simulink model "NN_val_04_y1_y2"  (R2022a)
settings: Solver=VariableStepAuto  StartTime=0.0  StopTime=300  RelTol=1e-3
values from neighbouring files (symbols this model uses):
  C = 6.3000e-04    (= 0.00063)    [maglev_init.m]
  g = 9.80    (= 9.8)    [maglev_init.m]
  K = 1.0e+03 * [-2.4567   -0.1235    0.0237]    [maglev_init.m]
  L1 = 0.6000    (= 0.6)    [maglev_init.m]
  m = 0.0300    (= 0.03)    [maglev_init.m]
  mpert = 0    [maglev_init.m]
  R = 45    [maglev_init.m]
  Ts = 0.005    [maglev_init.m]    (also in train_net.m)
  x1_0 = 0.1    [maglev_init.m]
  x1_d = 0.05    [maglev_init.m]
  x2_0 = 0    [maglev_init.m]
  x2_d = 0    [maglev_init.m]
  x3_0 = 0.2    [maglev_init.m]
undefined symbols (not defined in the file or in its folder): magnitude
libraries: neural x24

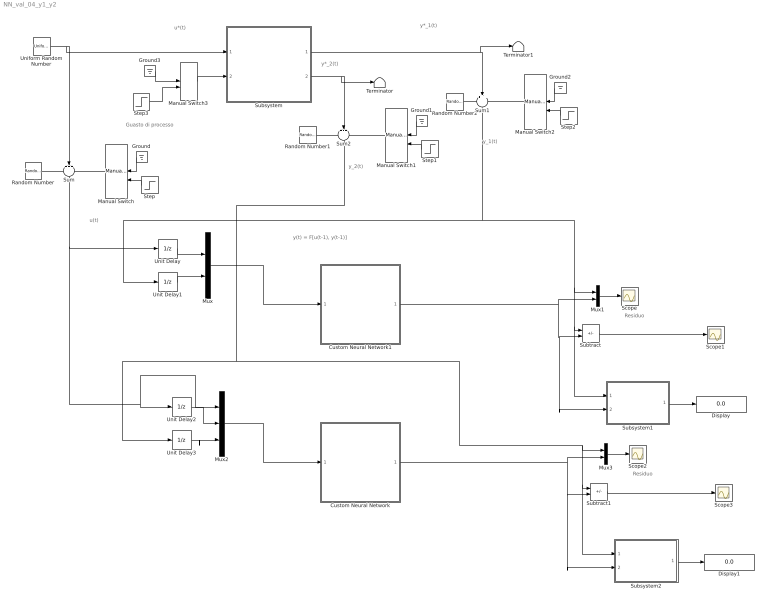
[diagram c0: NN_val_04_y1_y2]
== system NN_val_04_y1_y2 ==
  note: Residuo
  note: y(t) = F[u(t-1), y(t-1)]
  note: y_2(t)
  note: y*_1(t)
  note: u(t)
  note: y*_2(t)
  note: y_1(t)
  note: u*(t)
  note: Guasto di processo
  note: Residuo
  Custom Neural Network : Subsystem
      mask help: Custom Neural Network
  Custom Neural Network1 : Subsystem
      mask help: Custom Neural Network
  Display : Display
  Display1 : Display
  Ground{,1..3} (4 alike) : Ground
  Manual Switch : ManualSwitch
  Manual Switch1 : ManualSwitch  CurrentSetting=0
  Manual Switch2 : ManualSwitch
  Manual Switch3 : ManualSwitch
  Mux : Mux  Inputs=2
  Mux1 : Mux  Inputs=2
  Mux2 : Mux  Inputs=3
  Mux3 : Mux  Inputs=2
  Random Number : RandomNumber  Variance=1e-9  Seed=1  SampleTime=Ts
  Random Number1 : RandomNumber  Variance=1e-6  Seed=3  SampleTime=Ts
  Random Number2 : RandomNumber  Variance=1e-9  Seed=2  SampleTime=Ts
  Scope{,1..3} (4 alike) : Scope
  Step : Step  Time=150  SampleTime=0
  Step1 : Step  Time=150  SampleTime=0
  Step2 : Step  Time=150  SampleTime=0
  Step3 : Step  Time=15  After=2*R  SampleTime=0
  Subsystem : Subsystem
  Subsystem1 : Subsystem
  Subsystem2 : Subsystem
  Subtract : Sum  Inputs=+-
  Subtract1 : Sum  Inputs=+-
  Sum : Sum  Inputs=+++
  Sum1 : Sum  Inputs=+++
  Sum2 : Sum  Inputs=+++
  Terminator : Terminator
  Terminator1 : Terminator
  Uniform Random Number : UniformRandomNumber  Minimum=x1_d*0.9  Maximum=x1_d*1.1  Seed=1  SampleTime=0.5
  Unit Delay{,1..3} (4 alike) : UnitDelay  SampleTime=Ts  HasFrameUpgradeWarning=on
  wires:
  Subsystem/1(Out1) -> Terminator1/1, Sum1/2
  Subsystem/2(Out2) -> Terminator/1, Sum2/2
  Random Number/1 -> Sum/1
  Manual Switch/1 -> Sum/3
  Manual Switch2/1 -> Sum1/3
  Manual Switch1/1 -> Sum2/3
  Random Number1/1 -> Sum2/1
  Ground/1 -> Manual Switch/1
  Step/1 -> Manual Switch/2
  Ground1/1 -> Manual Switch1/1
  Step1/1 -> Manual Switch1/2
  Random Number2/1 -> Sum1/1
  Ground2/1 -> Manual Switch2/1
  Step2/1 -> Manual Switch2/2
  Manual Switch3/1 -> Subsystem/2(fs)
  Ground3/1 -> Manual Switch3/1
  Uniform Random Number/1 -> Subsystem/1(u), Sum/2
  Step3/1 -> Manual Switch3/2
  Sum/1 -> Mux2/1, Unit Delay2/1, Unit Delay/1
  Unit Delay/1 -> Mux/1
  Unit Delay1/1 -> Mux/2
  Mux/1 -> Custom Neural Network1/1(Input)
  Custom Neural Network1/1(Output) -> Mux1/2, Subsystem1/2(y_prev), Subtract/2
  Subtract/1 -> Scope1/1
  Mux1/1 -> Scope/1
  Sum1/1 -> Subsystem1/1(y_mis), Subtract/1, Mux1/1, Unit Delay1/1
  Subsystem1/1(VAF%) -> Display/1
  Mux2/1 -> Custom Neural Network/1(Input)
  Unit Delay2/1 -> Mux2/2
  Unit Delay3/1 -> Mux2/3
  Subtract1/1 -> Scope3/1
  Custom Neural Network/1(Output) -> Mux3/2, Subsystem2/2(y_prev), Subtract1/2
  Mux3/1 -> Scope2/1
  Subsystem2/1(VAF%) -> Display1/1
  Sum2/1 -> Subsystem2/1(y_mis), Subtract1/1, Mux3/1, Unit Delay3/1

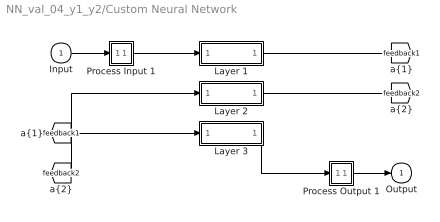
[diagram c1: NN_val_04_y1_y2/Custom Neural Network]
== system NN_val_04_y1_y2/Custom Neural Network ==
  Input : Inport  PortDimensions=3  SampleTime=0.005
  Layer 1 : Subsystem
  Layer 2 : Subsystem
  Layer 3 : Subsystem
  Process Input 1 : Subsystem
  Process Output 1 : Subsystem
  Output : Outport  InitialOutput=0
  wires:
  Input/1 -> Process Input 1/1(x)
  Process Output 1/1(y) -> Output/1
  Process Input 1/1(p) -> Layer 1/1("p{1}")
  Layer 1/1("a{1}") -> [feedback1]
  [feedback1] -> Layer 2/1("a{1} ")
  Layer 2/1("a{2}") -> [feedback2]
  [feedback2] -> Layer 3/1("a{2} ")
  Layer 3/1("a{3}") -> Process Output 1/1(a)

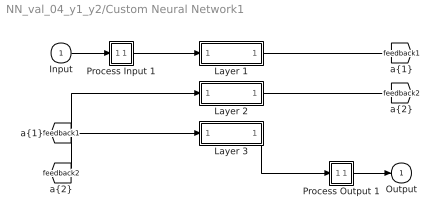
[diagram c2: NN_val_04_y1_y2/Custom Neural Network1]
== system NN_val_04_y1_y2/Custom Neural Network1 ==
  Input : Inport  PortDimensions=2  SampleTime=0.005
  Layer 1 : Subsystem
  Layer 2 : Subsystem
  Layer 3 : Subsystem
  Process Input 1 : Subsystem
  Process Output 1 : Subsystem
  Output : Outport  InitialOutput=0
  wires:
  Layer 3/1("a{3}") -> Process Output 1/1(a)
  [feedback2] -> Layer 3/1("a{2} ")
  Layer 2/1("a{2}") -> [feedback2]
  [feedback1] -> Layer 2/1("a{1} ")
  Layer 1/1("a{1}") -> [feedback1]
  Process Input 1/1(p) -> Layer 1/1("p{1}")
  Process Output 1/1(y) -> Output/1
  Input/1 -> Process Input 1/1(x)

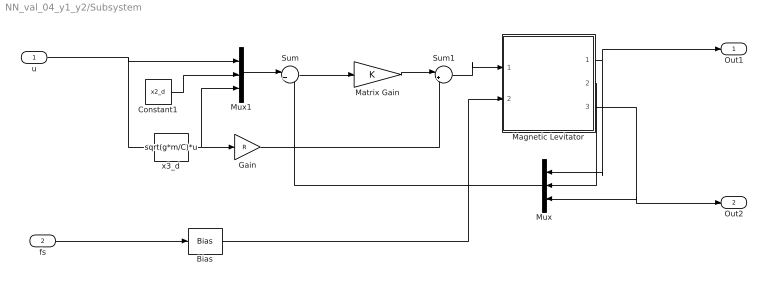
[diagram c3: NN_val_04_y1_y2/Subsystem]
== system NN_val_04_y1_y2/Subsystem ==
  u : Inport
  fs : Inport  Port=2
  Bias : Bias  Bias=R
  Constant1 : Constant  Value=x2_d
  Gain : Gain  Gain=R
  Magnetic Levitator : Subsystem  mask{m=m+mpert, R=R, L1=L1, C=C, g=g}
      mask prompts: m "ball's mass (m)"; R "Electromagnet's resistance (R)"; L1 "Electromagnet's inductance (L1)"; C "Magnetic force constant (C)"; g "Gravitational acceleration (g)"
  Matrix Gain : Gain  Gain=K  Multiplication=Matrix(K*u)  SaturateOnIntegerOverflow=on
  Mux : Mux  Inputs=3
  Mux1 : Mux  Inputs=3
  Sum : Sum  Inputs=|+-  InputSameDT=on  SaturateOnIntegerOverflow=on
  Sum1 : Sum  Inputs=|++  InputSameDT=on  SaturateOnIntegerOverflow=on
  x3_d : Fcn  Expr=sqrt(g*m/C)*u
  Out1 : Outport
  Out2 : Outport  Port=2
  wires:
  u/1 -> x3_d/1, Mux1/1
  Magnetic Levitator/2(x2) -> Mux/2
  x3_d/1 -> Mux1/3, Gain/1
  Mux1/1 -> Sum/1
  Gain/1 -> Sum1/2
  Mux/1 -> Sum/2
  Constant1/1 -> Mux1/2
  Sum/1 -> Matrix Gain/1
  Sum1/1 -> Magnetic Levitator/1(u)
  Magnetic Levitator/1(x1) -> Out1/1, Mux/1
  Magnetic Levitator/3(x3) -> Out2/1, Mux/3
  Matrix Gain/1 -> Sum1/1
  Bias/1 -> Magnetic Levitator/2(fs)
  fs/1 -> Bias/1

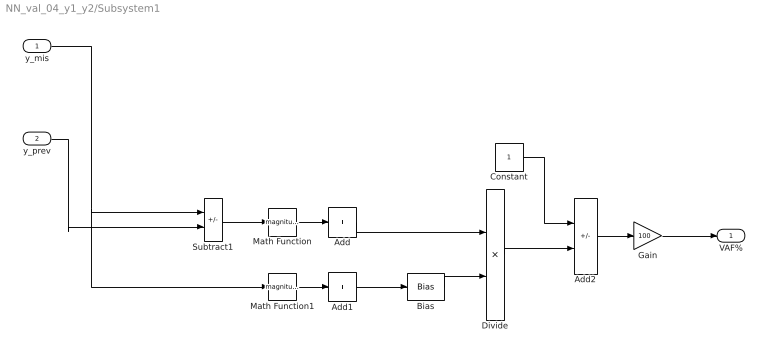
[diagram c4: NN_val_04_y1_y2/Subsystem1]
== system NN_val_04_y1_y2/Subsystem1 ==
  y_mis : Inport
  y_prev : Inport  Port=2
  Add : Sum  Inputs=+
  Add1 : Sum  Inputs=+
  Add2 : Sum  Inputs=+-
  Bias : Bias  Bias=1e-7
  Constant : Constant
  Divide : Product  Inputs=*/
  Gain : Gain  Gain=100
  Math Function : Math  Operator=magnitude^2
  Math Function1 : Math  Operator=magnitude^2
  Subtract1 : Sum  Inputs=+-
  VAF% : Outport
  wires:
  Add2/1 -> Gain/1
  Math Function/1 -> Add/1
  Bias/1 -> Divide/2
  y_mis/1 -> Math Function1/1, Subtract1/1
  Add1/1 -> Bias/1
  Math Function1/1 -> Add1/1
  Subtract1/1 -> Math Function/1
  Constant/1 -> Add2/1
  Divide/1 -> Add2/2
  Add/1 -> Divide/1
  y_prev/1 -> Subtract1/2
  Gain/1 -> VAF%/1

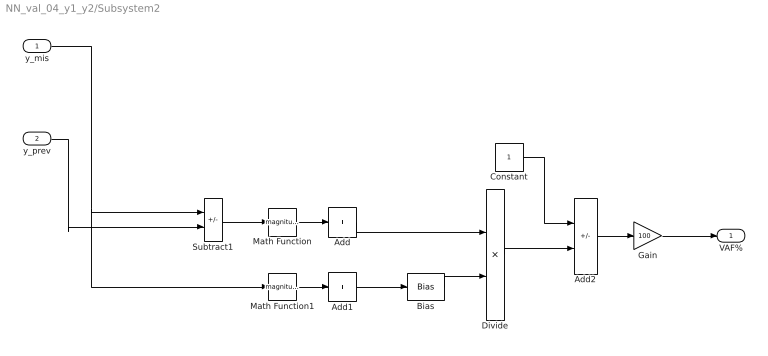
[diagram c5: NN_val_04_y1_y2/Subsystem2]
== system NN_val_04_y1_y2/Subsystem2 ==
  y_mis : Inport
  y_prev : Inport  Port=2
  Add : Sum  Inputs=+
  Add1 : Sum  Inputs=+
  Add2 : Sum  Inputs=+-
  Bias : Bias  Bias=1e-7
  Constant : Constant
  Divide : Product  Inputs=*/
  Gain : Gain  Gain=100
  Math Function : Math  Operator=magnitude^2
  Math Function1 : Math  Operator=magnitude^2
  Subtract1 : Sum  Inputs=+-
  VAF% : Outport
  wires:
  Add2/1 -> Gain/1
  Math Function/1 -> Add/1
  Bias/1 -> Divide/2
  y_mis/1 -> Math Function1/1, Subtract1/1
  Add1/1 -> Bias/1
  Math Function1/1 -> Add1/1
  Subtract1/1 -> Math Function/1
  Constant/1 -> Add2/1
  Divide/1 -> Add2/2
  Add/1 -> Divide/1
  y_prev/1 -> Subtract1/2
  Gain/1 -> VAF%/1

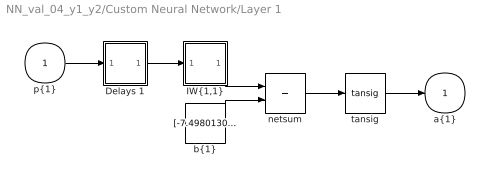
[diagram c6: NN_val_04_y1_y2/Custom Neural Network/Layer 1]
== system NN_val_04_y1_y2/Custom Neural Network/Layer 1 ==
  "p{1}" : Inport  PortDimensions=3  SampleTime=0.005
  Delays 1 : Subsystem
  "IW{1,1}" : Subsystem
  "b{1}" : Constant  Value=[-7.49801301032872391516548304934985935688018798828125;-8.469632793028239348132046870887279510498046875;-6.44515742607553843157575101940892636775970458984375]
  netsum : Sum  Inputs=2  InputSameDT=on  SaturateOnIntegerOverflow=on
  tansig : neural/Transfer Functions/tansig
  "a{1}" : Outport  InitialOutput=[0;0;0]
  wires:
  "p{1}"/1 -> Delays 1/1("p{1}")
  Delays 1/1("pd{1,1}") -> "IW{1,1}"/1("pd{1,1}")
  "IW{1,1}"/1("iz{1,1}") -> netsum/1
  "b{1}"/1 -> netsum/2
  netsum/1 -> tansig/1
  tansig/1 -> "a{1}"/1

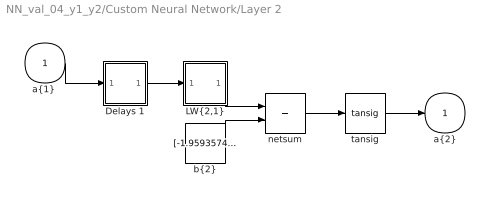
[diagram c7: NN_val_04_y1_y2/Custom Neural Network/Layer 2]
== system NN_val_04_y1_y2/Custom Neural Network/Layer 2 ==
  "a{1} " : Inport  PortDimensions=3  SampleTime=0.005
  Delays 1 : Subsystem
  "LW{2,1}" : Subsystem
  "b{2}" : Constant  Value=[-1.9593574661046309071110727018094621598720550537109375;-1.733772264384629835376472328789532184600830078125;-1.2022508025021882982485976754105649888515472412109375;0.15838977813118992887808644809410907328128814697265625;-0.346755044752183161360648000481887720525264739990234375;-1.1898913744646983925434824413969181478023529052734375;3.4402368274347878696062252856791019439697265625]
  netsum : Sum  Inputs=2  InputSameDT=on  SaturateOnIntegerOverflow=on
  tansig : neural/Transfer Functions/tansig
  "a{2}" : Outport  InitialOutput=[0;0;0;0;0;0;0]
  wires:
  "a{1} "/1 -> Delays 1/1("p{2}")
  Delays 1/1("pd{2,1}") -> "LW{2,1}"/1("ad{2,1}")
  "LW{2,1}"/1("lz{2,1}") -> netsum/1
  "b{2}"/1 -> netsum/2
  netsum/1 -> tansig/1
  tansig/1 -> "a{2}"/1

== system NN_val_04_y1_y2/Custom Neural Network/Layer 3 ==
  "a{2} " : Inport  PortDimensions=7  SampleTime=0.005
  Delays 1 : Subsystem
  "LW{3,2}" : Subsystem
  "b{3}" : Constant  Value=0.6308795893444221203338884151889942586421966552734375
  netsum : Sum  Inputs=2  InputSameDT=on  SaturateOnIntegerOverflow=on
  purelin : neural/Transfer Functions/purelin
  "a{3}" : Outport  InitialOutput=0
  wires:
  "a{2} "/1 -> Delays 1/1("p{3}")
  Delays 1/1("pd{3,2}") -> "LW{3,2}"/1("ad{3,2}")
  "LW{3,2}"/1("lz{3,2}") -> netsum/1
  "b{3}"/1 -> netsum/2
  netsum/1 -> purelin/1
  purelin/1 -> "a{3}"/1

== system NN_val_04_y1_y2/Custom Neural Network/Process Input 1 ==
  x : Inport  PortDimensions=3  SampleTime=0.005
  p : Outport  PortDimensions=3  SampleTime=0.005
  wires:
  x/1 -> p/1

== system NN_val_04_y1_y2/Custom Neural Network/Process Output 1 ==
  a : Inport  PortDimensions=1  SampleTime=0.005
  y : Outport  PortDimensions=1  SampleTime=0.005
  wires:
  a/1 -> y/1

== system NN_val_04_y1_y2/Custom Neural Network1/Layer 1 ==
  "p{1}" : Inport  PortDimensions=2  SampleTime=0.005
  Delays 1 : Subsystem
  "IW{1,1}" : Subsystem
  "b{1}" : Constant  Value=[-2.165010232984565075042837634100578725337982177734375;-0.99018084463472033629471980020753107964992523193359375]
  netsum : Sum  Inputs=2  InputSameDT=on  SaturateOnIntegerOverflow=on
  tansig : neural/Transfer Functions/tansig
  "a{1}" : Outport  InitialOutput=[0;0]
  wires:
  tansig/1 -> "a{1}"/1
  netsum/1 -> tansig/1
  "b{1}"/1 -> netsum/2
  "IW{1,1}"/1("iz{1,1}") -> netsum/1
  Delays 1/1("pd{1,1}") -> "IW{1,1}"/1("pd{1,1}")
  "p{1}"/1 -> Delays 1/1("p{1}")

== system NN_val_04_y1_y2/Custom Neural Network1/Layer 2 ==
  "a{1} " : Inport  PortDimensions=2  SampleTime=0.005
  Delays 1 : Subsystem
  "LW{2,1}" : Subsystem
  "b{2}" : Constant  Value=[-2.76409742947160541604034733609296381473541259765625;0.91391405324340713178798978333361446857452392578125;-0.79693396570784413857069239384145475924015045166015625;2.83340357653886432132139816530980169773101806640625]
  netsum : Sum  Inputs=2  InputSameDT=on  SaturateOnIntegerOverflow=on
  tansig : neural/Transfer Functions/tansig
  "a{2}" : Outport  InitialOutput=[0;0;0;0]
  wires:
  tansig/1 -> "a{2}"/1
  netsum/1 -> tansig/1
  "b{2}"/1 -> netsum/2
  "LW{2,1}"/1("lz{2,1}") -> netsum/1
  Delays 1/1("pd{2,1}") -> "LW{2,1}"/1("ad{2,1}")
  "a{1} "/1 -> Delays 1/1("p{2}")

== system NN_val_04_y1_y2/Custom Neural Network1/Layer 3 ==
  "a{2} " : Inport  PortDimensions=4  SampleTime=0.005
  Delays 1 : Subsystem
  "LW{3,2}" : Subsystem
  "b{3}" : Constant  Value=0.2010605623167778244209102922468446195125579833984375
  netsum : Sum  Inputs=2  InputSameDT=on  SaturateOnIntegerOverflow=on
  purelin : neural/Transfer Functions/purelin
  "a{3}" : Outport  InitialOutput=0
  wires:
  purelin/1 -> "a{3}"/1
  netsum/1 -> purelin/1
  "b{3}"/1 -> netsum/2
  "LW{3,2}"/1("lz{3,2}") -> netsum/1
  Delays 1/1("pd{3,2}") -> "LW{3,2}"/1("ad{3,2}")
  "a{2} "/1 -> Delays 1/1("p{3}")

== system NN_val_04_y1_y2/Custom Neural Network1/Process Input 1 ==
  x : Inport  PortDimensions=2  SampleTime=0.005
  p : Outport  PortDimensions=2  SampleTime=0.005
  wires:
  x/1 -> p/1

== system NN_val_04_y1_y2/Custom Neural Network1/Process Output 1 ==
  a : Inport  PortDimensions=1  SampleTime=0.005
  y : Outport  PortDimensions=1  SampleTime=0.005
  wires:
  a/1 -> y/1

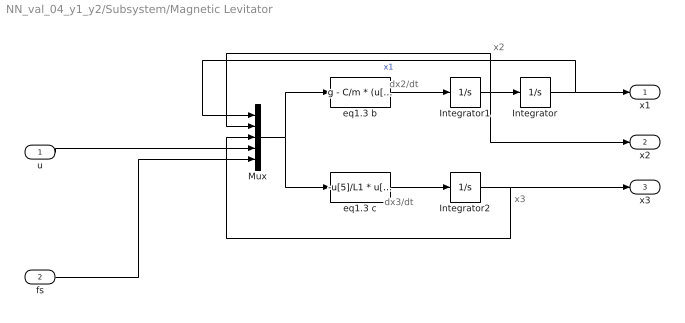
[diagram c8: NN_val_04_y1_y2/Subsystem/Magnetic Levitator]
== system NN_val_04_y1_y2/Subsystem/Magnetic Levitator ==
  note: x2
  note: x3
  note: dx2/dt
  note: dx3/dt
  u : Inport
  fs : Inport  Port=2
  Integrator : Integrator  InitialCondition=x1_0
  Integrator1 : Integrator  InitialCondition=x2_0
  Integrator2 : Integrator  InitialCondition=x3_0
  Mux : Mux  Inputs=5
  eq1.3 b : Fcn  Expr=g - C/m * (u[3] / u[1])^2
  eq1.3 c : Fcn  Expr=-u[5]/L1 * u[3] + (2*C)/L1 * ( u[2] * u[3] / u[1]^2 ) + 1/L1 * u[4]
  x1 : Outport
  x2 : Outport  Port=2
  x3 : Outport  Port=3
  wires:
  eq1.3 b/1 -> Integrator1/1
  Integrator1/1 -> Integrator/1, Mux/2, x2/1
  eq1.3 c/1 -> Integrator2/1
  Mux/1 -> eq1.3 b/1, eq1.3 c/1
  Integrator/1 -> Mux/1, x1/1  "x1"
  Integrator2/1 -> Mux/3, x3/1
  u/1 -> Mux/4
  fs/1 -> Mux/5

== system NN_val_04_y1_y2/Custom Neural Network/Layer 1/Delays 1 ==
  "p{1}" : Inport  PortDimensions=3  SampleTime=0.005
  mux : Mux  Inputs=1
  "pd{1,1}" : Outport
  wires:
  "p{1}"/1 -> mux/1
  mux/1 -> "pd{1,1}"/1

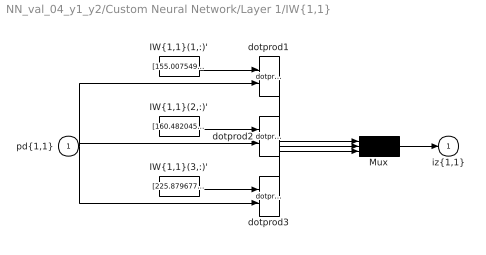
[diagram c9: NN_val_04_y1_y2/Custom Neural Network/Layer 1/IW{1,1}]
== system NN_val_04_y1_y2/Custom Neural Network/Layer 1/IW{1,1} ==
  "pd{1,1}" : Inport  PortDimensions=3  SampleTime=0.005
  "IW{1,1}(1,:)'" : Constant  Value=[155.0075492278721185357426293194293975830078125;-67.6206153138385843703872524201869964599609375;-1.56484201084633678391355715575627982616424560546875]
  "IW{1,1}(2,:)'" : Constant  Value=[160.482045237883454547045403160154819488525390625;-62.3839210025603989606679533608257770538330078125;3.692954814299637344987559117726050317287445068359375]
  "IW{1,1}(3,:)'" : Constant  Value=[225.879677595525521383024170063436031341552734375;-54.79104188249477402905540657229721546173095703125;-1.4456599193376373779784671569359488785266876220703125]
  Mux : Mux  Inputs=3
  dotprod1 : neural/Weight Functions/dotprod
  dotprod2 : neural/Weight Functions/dotprod
  dotprod3 : neural/Weight Functions/dotprod
  "iz{1,1}" : Outport
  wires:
  "IW{1,1}(1,:)'"/1 -> dotprod1/1
  "pd{1,1}"/1 -> dotprod1/2, dotprod2/2, dotprod3/2
  dotprod1/1 -> Mux/1
  "IW{1,1}(2,:)'"/1 -> dotprod2/1
  dotprod2/1 -> Mux/2
  "IW{1,1}(3,:)'"/1 -> dotprod3/1
  dotprod3/1 -> Mux/3
  Mux/1 -> "iz{1,1}"/1

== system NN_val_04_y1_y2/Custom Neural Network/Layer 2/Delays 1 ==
  "p{2}" : Inport  PortDimensions=3  SampleTime=0.005
  mux : Mux  Inputs=1
  "pd{2,1}" : Outport
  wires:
  "p{2}"/1 -> mux/1
  mux/1 -> "pd{2,1}"/1

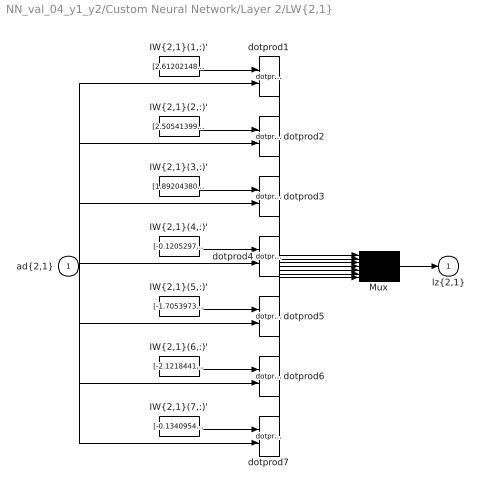
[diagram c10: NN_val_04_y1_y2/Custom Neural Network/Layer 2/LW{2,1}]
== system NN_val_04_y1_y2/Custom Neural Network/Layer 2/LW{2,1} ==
  "ad{2,1}" : Inport  PortDimensions=3  SampleTime=0.005
  "IW{2,1}(1,:)'" : Constant  Value=[2.61202148304921966115443865419365465641021728515625;0.14862508312520861242234104793169535696506500244140625;2.66275173354789185253821415244601666927337646484375]
  "IW{2,1}(2,:)'" : Constant  Value=[2.505413996791865383073627526755444705486297607421875;-0.87551618416646681541948282756493426859378814697265625;-0.4467990015803449121989388004294596612453460693359375]
  "IW{2,1}(3,:)'" : Constant  Value=[1.8920438003690247530386159269255585968494415283203125;-2.18523469881069587472666171379387378692626953125;0.99273270475465125173286651261150836944580078125]
  "IW{2,1}(4,:)'" : Constant  Value=[-0.12052978882303892749217055779809015803039073944091796875;-1.505868112384237900158723277854733169078826904296875;-0.009347378292273882116614203141580219380557537078857421875]
  "IW{2,1}(5,:)'" : Constant  Value=[-1.70539739975583959363802932784892618656158447265625;-2.30803401714740186179142256150953471660614013671875;0.43818271298305833116870644516893662512302398681640625]
  "IW{2,1}(6,:)'" : Constant  Value=[-2.12184410470687101479825287242420017719268798828125;-0.95495157641803307679850831846124492585659027099609375;0.1571940959909395030269507742559653706848621368408203125]
  "IW{2,1}(7,:)'" : Constant  Value=[-0.1340954916262217244682375394404516555368900299072265625;-0.33392737163233976449561168919899500906467437744140625;2.924572272947035589396591603872366249561309814453125]
  Mux : Mux  Inputs=7
  dotprod{1..7} (7 alike) : neural/Weight Functions/dotprod
  "lz{2,1}" : Outport
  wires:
  "IW{2,1}(1,:)'"/1 -> dotprod1/1
  "ad{2,1}"/1 -> dotprod1/2, dotprod2/2, dotprod3/2, dotprod4/2, dotprod5/2, dotprod6/2, dotprod7/2
  dotprod1/1 -> Mux/1
  "IW{2,1}(2,:)'"/1 -> dotprod2/1
  dotprod2/1 -> Mux/2
  "IW{2,1}(3,:)'"/1 -> dotprod3/1
  dotprod3/1 -> Mux/3
  "IW{2,1}(4,:)'"/1 -> dotprod4/1
  dotprod4/1 -> Mux/4
  "IW{2,1}(5,:)'"/1 -> dotprod5/1
  dotprod5/1 -> Mux/5
  "IW{2,1}(6,:)'"/1 -> dotprod6/1
  dotprod6/1 -> Mux/6
  "IW{2,1}(7,:)'"/1 -> dotprod7/1
  dotprod7/1 -> Mux/7
  Mux/1 -> "lz{2,1}"/1

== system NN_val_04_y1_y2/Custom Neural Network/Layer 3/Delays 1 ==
  "p{3}" : Inport  PortDimensions=7  SampleTime=0.005
  mux : Mux  Inputs=1
  "pd{3,2}" : Outport
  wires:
  "p{3}"/1 -> mux/1
  mux/1 -> "pd{3,2}"/1

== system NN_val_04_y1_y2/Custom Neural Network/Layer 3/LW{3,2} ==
  "ad{3,2}" : Inport  PortDimensions=7  SampleTime=0.005
  "IW{3,2}(1,:)'" : Constant  Value=[-2.790612652168341423219999342109076678752899169921875;-0.8765399083285443371238443432957865297794342041015625;0.59844685053375357153271352217416279017925262451171875;0.355938703295180236541028762076166458427906036376953125;0.46820214887316835561392736053676344454288482666015625;-2.2275650588955588915496264235116541385650634765625;-1.5266001776393240962903519175597466528415679931640625]
  Mux : Mux  Inputs=1
  dotprod1 : neural/Weight Functions/dotprod
  "lz{3,2}" : Outport
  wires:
  "IW{3,2}(1,:)'"/1 -> dotprod1/1
  "ad{3,2}"/1 -> dotprod1/2
  dotprod1/1 -> Mux/1
  Mux/1 -> "lz{3,2}"/1

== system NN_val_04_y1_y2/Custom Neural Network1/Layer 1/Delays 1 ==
  "p{1}" : Inport  PortDimensions=2  SampleTime=0.005
  mux : Mux  Inputs=1
  "pd{1,1}" : Outport
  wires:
  mux/1 -> "pd{1,1}"/1
  "p{1}"/1 -> mux/1

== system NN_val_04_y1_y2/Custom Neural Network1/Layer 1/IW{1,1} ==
  "pd{1,1}" : Inport  PortDimensions=2  SampleTime=0.005
  "IW{1,1}(1,:)'" : Constant  Value=[46.38752532641807846403025905601680278778076171875;-30.02020716206245509738437249325215816497802734375]
  "IW{1,1}(2,:)'" : Constant  Value=[50.408506029134514392353594303131103515625;28.00458439829532153453328646719455718994140625]
  Mux : Mux  Inputs=2
  dotprod1 : neural/Weight Functions/dotprod
  dotprod2 : neural/Weight Functions/dotprod
  "iz{1,1}" : Outport
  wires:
  Mux/1 -> "iz{1,1}"/1
  dotprod2/1 -> Mux/2
  "IW{1,1}(2,:)'"/1 -> dotprod2/1
  dotprod1/1 -> Mux/1
  "pd{1,1}"/1 -> dotprod2/2, dotprod1/2
  "IW{1,1}(1,:)'"/1 -> dotprod1/1

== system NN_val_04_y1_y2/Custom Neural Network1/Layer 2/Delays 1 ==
  "p{2}" : Inport  PortDimensions=2  SampleTime=0.005
  mux : Mux  Inputs=1
  "pd{2,1}" : Outport
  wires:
  mux/1 -> "pd{2,1}"/1
  "p{2}"/1 -> mux/1

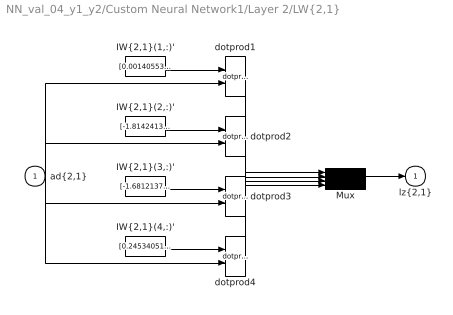
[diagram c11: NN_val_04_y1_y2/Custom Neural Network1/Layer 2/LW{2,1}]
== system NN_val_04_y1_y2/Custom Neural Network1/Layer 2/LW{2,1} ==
  "ad{2,1}" : Inport  PortDimensions=2  SampleTime=0.005
  "IW{2,1}(1,:)'" : Constant  Value=[0.001405533007920074795027431946436990983784198760986328125;2.76441434699151766807290186989121139049530029296875]
  "IW{2,1}(2,:)'" : Constant  Value=[-1.8142413042354241792253333187545649707317352294921875;2.12830136073460085555097975884564220905303955078125]
  "IW{2,1}(3,:)'" : Constant  Value=[-1.6812137832937150694334604850155301392078399658203125;-2.2096304124726291462366134510375559329986572265625]
  "IW{2,1}(4,:)'" : Constant  Value=[0.245340519136751533668672209387295879423618316650390625;2.76382363851122736519982936442829668521881103515625]
  Mux : Mux
  dotprod{1..4} (4 alike) : neural/Weight Functions/dotprod
  "lz{2,1}" : Outport
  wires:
  Mux/1 -> "lz{2,1}"/1
  dotprod4/1 -> Mux/4
  "IW{2,1}(4,:)'"/1 -> dotprod4/1
  dotprod3/1 -> Mux/3
  "IW{2,1}(3,:)'"/1 -> dotprod3/1
  dotprod2/1 -> Mux/2
  "IW{2,1}(2,:)'"/1 -> dotprod2/1
  dotprod1/1 -> Mux/1
  "ad{2,1}"/1 -> dotprod4/2, dotprod3/2, dotprod2/2, dotprod1/2
  "IW{2,1}(1,:)'"/1 -> dotprod1/1

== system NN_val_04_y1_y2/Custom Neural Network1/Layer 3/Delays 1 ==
  "p{3}" : Inport  PortDimensions=4  SampleTime=0.005
  mux : Mux  Inputs=1
  "pd{3,2}" : Outport
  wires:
  mux/1 -> "pd{3,2}"/1
  "p{3}"/1 -> mux/1

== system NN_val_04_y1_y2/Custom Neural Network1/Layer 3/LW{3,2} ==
  "ad{3,2}" : Inport  PortDimensions=4  SampleTime=0.005
  "IW{3,2}(1,:)'" : Constant  Value=[0.483295609205659226770279701668187044560909271240234375;0.356104986175123150449195463806972838938236236572265625;0.2319393811096205626487432027715840376913547515869140625;-0.2873034152097859728058892869739793241024017333984375]
  Mux : Mux  Inputs=1
  dotprod1 : neural/Weight Functions/dotprod
  "lz{3,2}" : Outport
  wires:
  Mux/1 -> "lz{3,2}"/1
  dotprod1/1 -> Mux/1
  "ad{3,2}"/1 -> dotprod1/2
  "IW{3,2}(1,:)'"/1 -> dotprod1/1
